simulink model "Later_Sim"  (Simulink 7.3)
settings: Solver=ode45  StartTime=0.0  StopTime=100  RelTol=1e-3
undefined symbols (not defined in the file or in its folder): Ad, Bd, Cd, Dd, Kpr

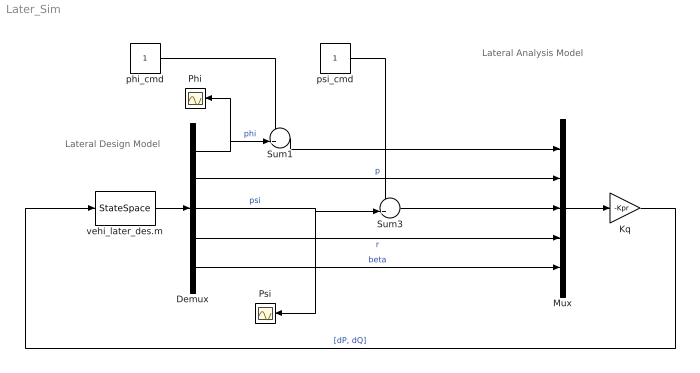
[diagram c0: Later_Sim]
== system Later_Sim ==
  note: Lateral Analysis Model
  note: Lateral Design Model
  Demux : Demux  Outputs=5
  Kq : Gain  Gain=-Kpr  Multiplication=Matrix(K*u) (u vector)  ParameterDataType=fixdt(1, 16)  ParameterScaling=2^0  OutDataType=fixdt(1, 16)  OutScaling=2^0
  Mux : Mux  Inputs=5
  Phi : Scope
  Psi : Scope
  Sum1 : Sum  Inputs=-+|  OutDataType=sfix(16)  OutScaling=2^0
  Sum3 : Sum  Inputs=-+|  OutDataType=sfix(16)  OutScaling=2^0
  phi_cmd : Constant  OutDataType=fixdt(1, 16)  OutScaling=2^0
  psi_cmd : Constant  OutDataType=fixdt(1, 16)  OutScaling=2^0
  vehi_later_des.m : StateSpace  A=Ad  B=Bd  C=Cd  D=Dd
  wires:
  vehi_later_des.m/1 -> Demux/1
  Kq/1 -> vehi_later_des.m/1  "[dP, dQ]"
  phi_cmd/1 -> Sum1/1
  Mux/1 -> Kq/1
  Demux/2 -> Mux/2  "p"
  Demux/4 -> Mux/4  "r"
  Demux/5 -> Mux/5  "beta"
  Demux/1 -> Sum1/2, Phi/1  "phi"
  Sum1/1 -> Mux/1
  Demux/3 -> Sum3/2, Psi/1  "psi"
  Sum3/1 -> Mux/3
  psi_cmd/1 -> Sum3/1
